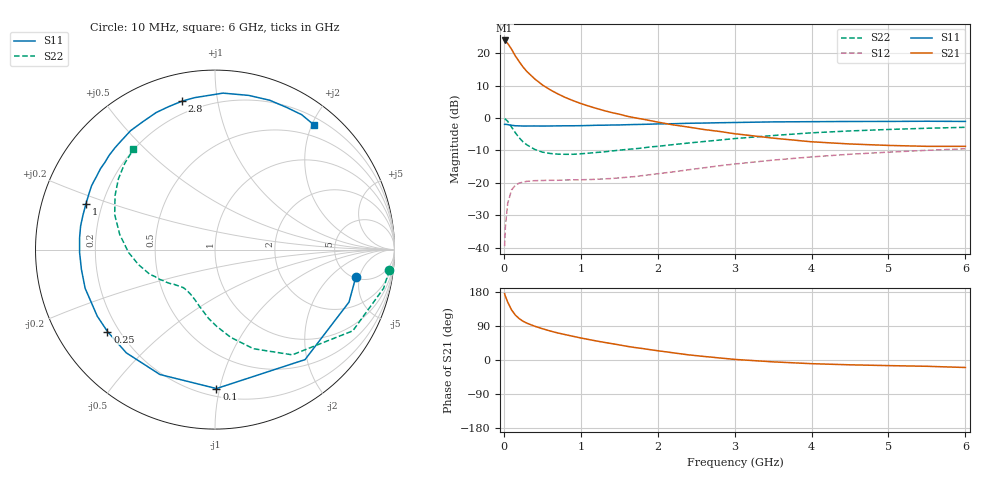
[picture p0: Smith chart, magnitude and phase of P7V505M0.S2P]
! SIEMENS Small Signal Semiconductors
! BFP196
! Si NPN RF Bipolar Junction Transistor in SOT143
! VCE = 0.5 V  IC = 5 mA
! Common Emitter S-Parameters:  May  1996
# GHz  S  MA  R  50
!  f  S11  S21  S12  S22
! GHz  MAG  ANG  MAG  ANG  MAG  ANG  MAG  ANG
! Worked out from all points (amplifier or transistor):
!   36 points, 10 MHz to 6 GHz, reference 50 ohm
!   highest |S21| = 24.0 dB at 10 MHz (marker M1)
!   |S21| within 3 dB of that: start of sweep to 107.1 MHz
!   unconditionally stable (mu >= 1): 1.037 GHz to end of sweep
!   at 250 MHz: K = 0.27, MSG = 17.8 dB, |S12| = -19.8 dB
!   at 1.4 GHz: K = 1.20, MAG = 7.5 dB, |S12| = -18.7 dB
!   at 6 GHz: K = 1.06, MAG = -1.1 dB, |S12| = -9.5 dB
!   S11 on the Smith chart (normalised r, x): 10 MHz: 5.15, -4.38; 100 MHz: 0.25, -0.98; 250 MHz: 0.16, -0.33; 1 GHz: 0.14, +0.17; 2.8 GHz: 0.14, +0.79; 6 GHz: 0.31, +2.03
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0.01  0.7993 -11.1  15.81 175.2  0.0105 84.7  0.9776 -6.7
0.02  0.8019 -21.4  15.3 168.3  0.021 78.9  0.9639 -12.9
0.05  0.7921 -50.7  14.24 152.7  0.048 64.0  0.8914 -30.5
0.1  0.7742 -89.4  11.58 132.3  0.0774 46.7  0.7275 -53.7
0.15  0.7606 -113.8  9.093 118.5  0.092 35.6  0.5924 -68.8
0.2  0.7584 -130.7  7.44 109.1  0.099 28.9  0.4963 -79.9
0.25  0.7532 -142.7  6.138 102.2  0.1025 24.5  0.428 -88.7
0.3  0.7536 -150.5  5.231 97.2  0.1054 21.9  0.3854 -95.3
0.4  0.755 -163.4  4.041 89.2  0.1079 18.1  0.3287 -105.1
0.5  0.7524 -171.6  3.26 82.6  0.1086 16.1  0.2982 -112.7
0.6  0.7547 -178.9  2.742 76.7  0.1093 15.7  0.284 -118.4
0.7  0.7574 174.9  2.369 71.4  0.1094 15.2  0.2775 -123.1
0.8  0.7601 170.1  2.078 66.9  0.1104 15.4  0.2756 -126.6
1  0.763 160.4  1.678 58.1  0.1114 16.9  0.2805 -132.5
1.1  0.7677 156.3  1.536 54.2  0.1123 17.9  0.2869 -135.2
1.6  0.7898 138.3  1.069 36.2  0.1218 23.8  0.3279 -146.6
2.2  0.8181 119.4  0.785 19.0  0.1474 28.9  0.3889 -159.3
2.8  0.8471 102.6  0.622 5.5  0.183 28.6  0.4572 -173.8
3.5  0.8729 87.1  0.49 -4.9  0.2242 23.2  0.5374 171.0
4.5  0.8862 69.9  0.398 -12.7  0.2762 12.6  0.6326 151.7
5.5  0.8934 57.3  0.366 -16.6  0.3177 1.5  0.696 136.2
6  0.8869 51.5  0.366 -19.8  0.3351 -4.5  0.7201 129.1
